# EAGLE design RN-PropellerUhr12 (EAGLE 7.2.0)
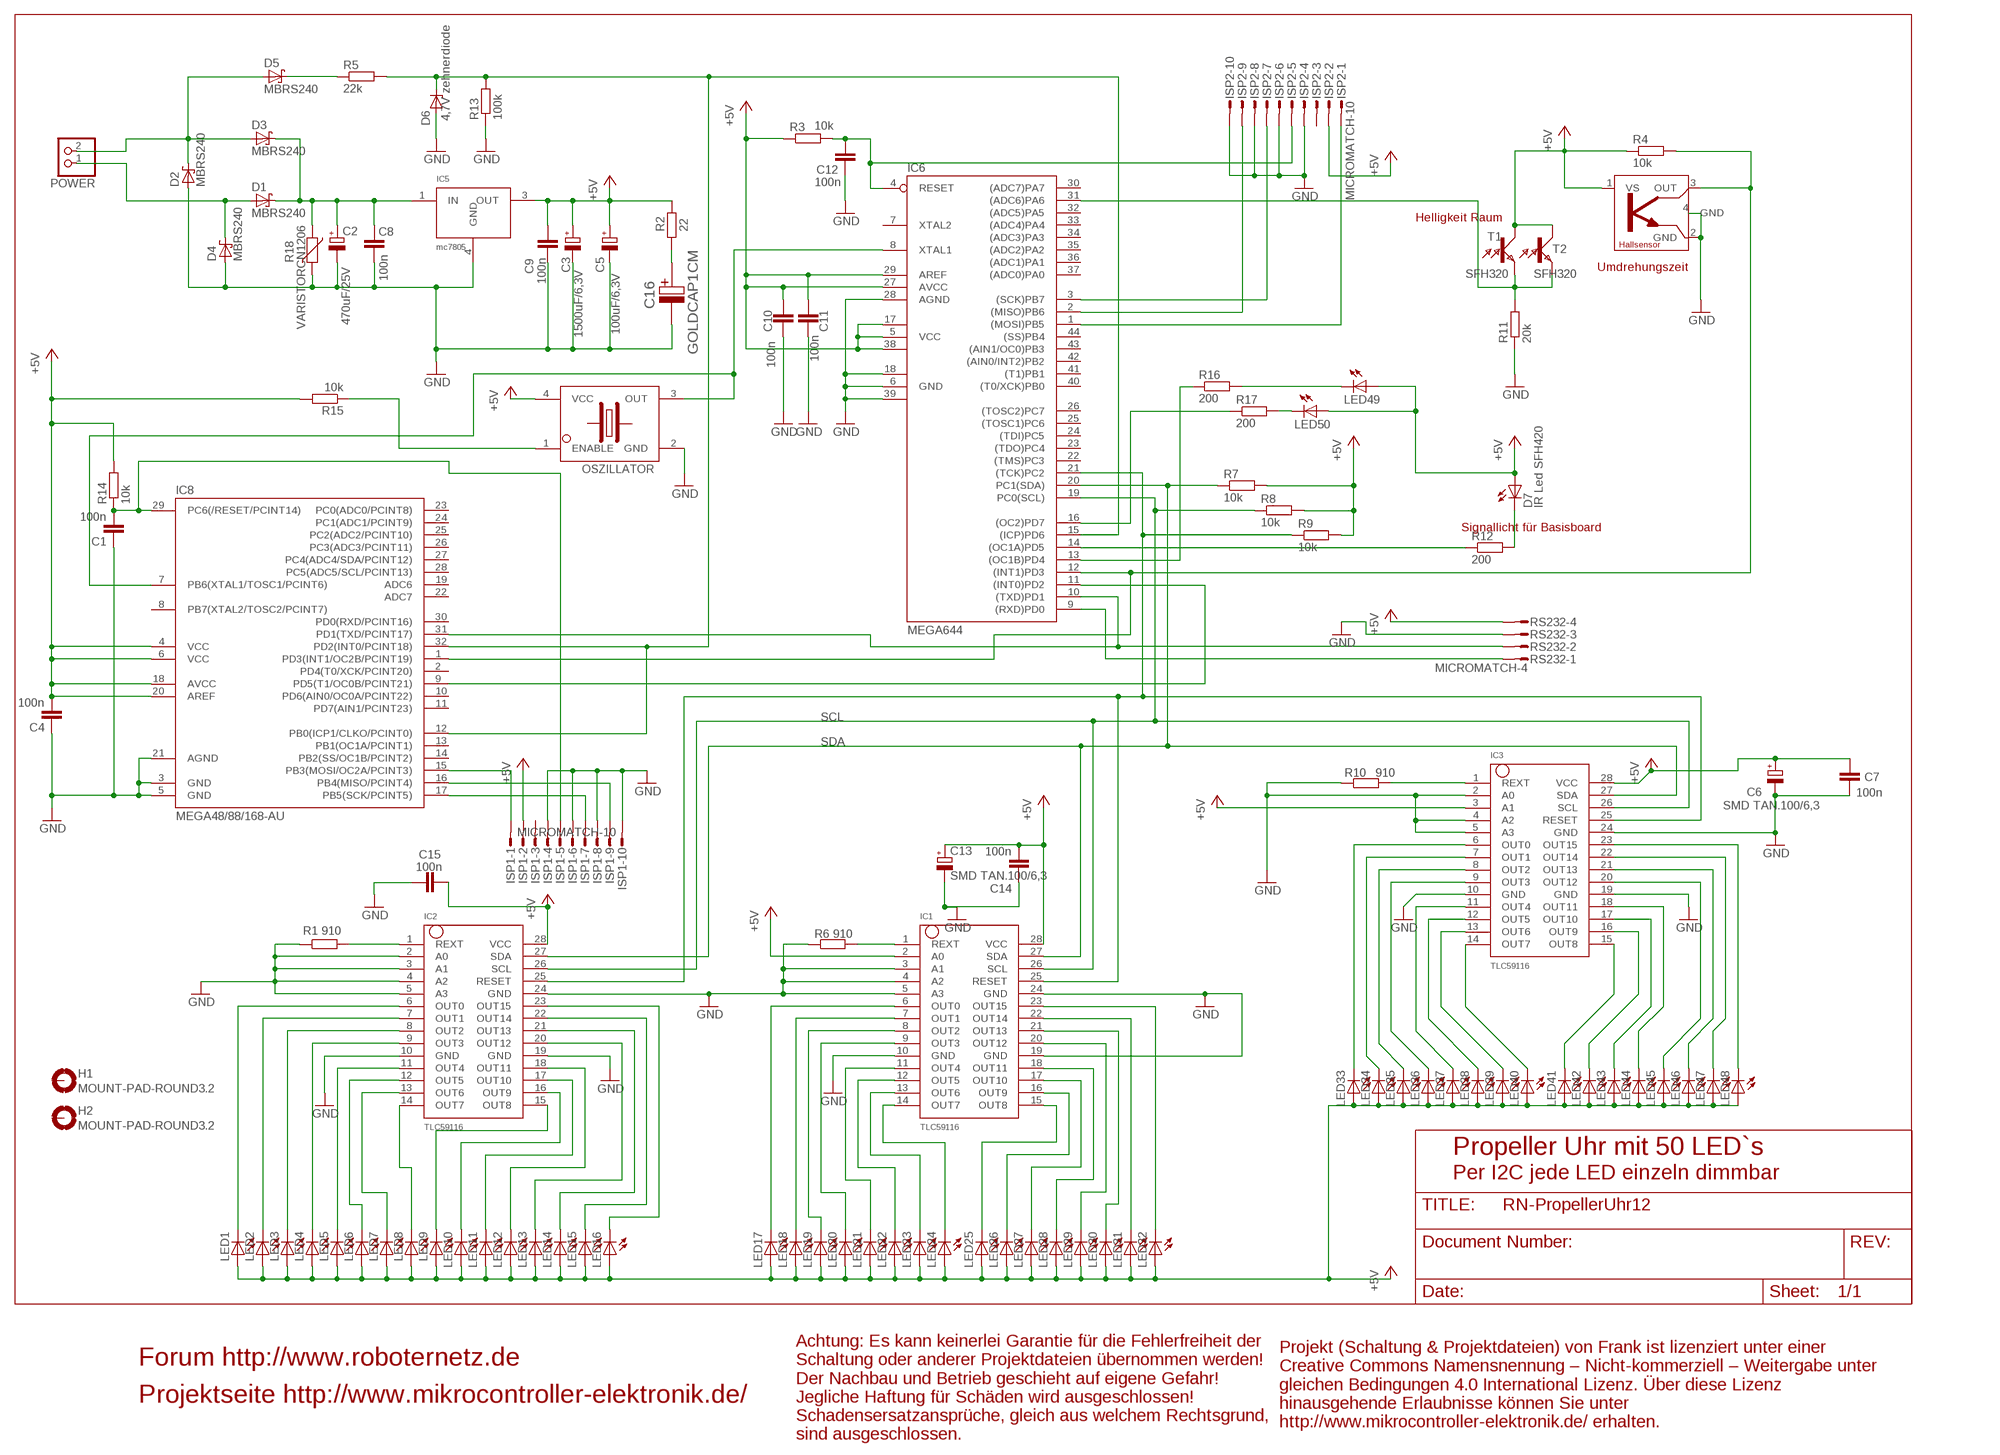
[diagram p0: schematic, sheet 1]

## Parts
C1  100n  C-EUC1206  [C1206]
C2  470uF/25V  CPOL-EU153CLV-1014  [153CLV-1014]
C3  1500uF/6,3V  CPOL-EU153CLV-1014  [153CLV-1014]
C4  100n  C-EUC1206  [C1206]
C5  100uF/6,3V  CPOL-EU153CLV-0605  [153CLV-0605]
C6  SMD TAN.100/6,3  CPOL-EUSMCD  [SMC_D]
C7  100n  C-EUC1206  [C1206]
C8  100n  C-EUC1206  [C1206]
C9  100n  C-EUC1206  [C1206]
C10  100n  C-EUC1206  [C1206]
C11  100n  C-EUC1206  [C1206]
C12  100n  C-EUC1206  [C1206]
C13  SMD TAN.100/6,3  CPOL-EUSMCD  [SMC_D]
C14  100n  C-EUC1206  [C1206]
C15  100n  C-EUC1206  [C1206]
C16  GOLDCAP1CM  [GOLDCAP10MM]
D1  MBRS240  [SMB]
D2  MBRS240  [SMB]
D3  MBRS240  [SMB]
D4  MBRS240  [SMB]
D5  MBRS240  [SMB]
D6  4,7V zehnerdiode  ZENER-DIODESOT23  [SOT23]
D7  IR Led SFH420  SFH420_IRLED  [OSRAM_SFH320]
H1  MOUNT-PAD-ROUND3.2  [3,2-PAD]
H2  MOUNT-PAD-ROUND3.2  [3,2-PAD]
IC1  TLC59116  [PW_R-PDSO-G28]
IC2  TLC59116  [PW_R-PDSO-G28]
IC3  TLC59116  [PW_R-PDSO-G28]
IC5  mc7805  MC7805  [DPAK]
IC6  MEGA644  MEGA32-A  [TQFP44]
IC7  TLE4905  TLE4905SOT89  [SOT89]
IC8  MEGA48/88/168-AU  [TQFP32-08]
ISP1  MICROMATCH-10  [MICROMATCH-10]
ISP2  MICROMATCH-10  [MICROMATCH-10]
LED1  LEDSMT1206  [1206]
LED2  LEDSMT1206  [1206]
LED3  LEDSMT1206  [1206]
LED4  LEDSMT1206  [1206]
LED5  LEDSMT1206  [1206]
LED6  LEDSMT1206  [1206]
LED7  LEDSMT1206  [1206]
LED8  LEDSMT1206  [1206]
LED9  LEDSMT1206  [1206]
LED10  LEDSMT1206  [1206]
LED11  LEDSMT1206  [1206]
LED12  LEDSMT1206  [1206]
LED13  LEDSMT1206  [1206]
LED14  LEDSMT1206  [1206]
LED15  LEDSMT1206  [1206]
LED16  LEDSMT1206  [1206]
LED17  LEDSMT1206  [1206]
LED18  LEDSMT1206  [1206]
LED19  LEDSMT1206  [1206]
LED20  LEDSMT1206  [1206]
LED21  LEDSMT1206  [1206]
LED22  LEDSMT1206  [1206]
LED23  LEDSMT1206  [1206]
LED24  LEDSMT1206  [1206]
LED25  LEDSMT1206  [1206]
LED26  LEDSMT1206  [1206]
LED27  LEDSMT1206  [1206]
LED28  LEDSMT1206  [1206]
LED29  LEDSMT1206  [1206]
LED30  LEDSMT1206  [1206]
LED31  LEDSMT1206  [1206]
LED32  LEDSMT1206  [1206]
LED33  LEDSMT1206  [1206]
LED34  LEDSMT1206  [1206]
LED35  LEDSMT1206  [1206]
LED36  LEDSMT1206  [1206]
LED37  LEDSMT1206  [1206]
LED38  LEDSMT1206  [1206]
LED39  LEDSMT1206  [1206]
LED40  LEDSMT1206  [1206]
LED41  LEDSMT1206  [1206]
LED42  LEDSMT1206  [1206]
LED43  LEDSMT1206  [1206]
LED44  LEDSMT1206  [1206]
LED45  LEDSMT1206  [1206]
LED46  LEDSMT1206  [1206]
LED47  LEDSMT1206  [1206]
LED48  LEDSMT1206  [1206]
LED49  LEDSMT1206  [1206]
LED50  LEDSMT1206  [1206]
OSZILLATOR  OSZILLATOR_AQO7050  [QUARZOSZILLATOR_AQO7050]
POWER  PINHD-1X2  [1X02]
R1  910  R-EU_M1206  [M1206]
R2  22  R-EU_M1206  [M1206]
R3  10k  R-EU_M1206  [M1206]
R4  10k  R-EU_M1206  [M1206]
R5  22k  R-EU_M1206  [M1206]
R6  910  R-EU_M1206  [M1206]
R7  10k  R-EU_M1206  [M1206]
R8  10k  R-EU_M1206  [M1206]
R9  10k  R-EU_M1206  [M1206]
R10  910  R-EU_M1206  [M1206]
R11  20k  R-EU_M1206  [M1206]
R12  200  R-EU_M1206  [M1206]
R13  100k  R-EU_M1206  [M1206]
R14  10k  R-EU_M1206  [M1206]
R15  10k  R-EU_M1206  [M1206]
R16  200  R-EU_M1206  [M1206]
R17  200  R-EU_M1206  [M1206]
R18  VARISTORCN1206  [CT/CN1206]
RS232  MICROMATCH-4  [MICROMATCH-4]
T1  SFH320  [OSRAM_SFH320]
T2  SFH320  [OSRAM_SFH320]

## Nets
+5V [Power]: C3.+ C4.2 C5.+ C6.+ C7.2 C9.2 C10.2 C11.2 C13.+ C14.2 C15.1 D7.E(A) IC1.2(A0) IC1.28(VCC) IC2.28(VCC) IC3.3(A1) IC3.28(VCC) IC5.3(OUT) IC6.5(VCC) IC6.17(VCC1) IC6.27(AVCC) IC6.29(AREF) IC6.38(VCC2) IC7.1(VS) IC8.4(VCC) IC8.6(VCC) IC8.18(AVCC) IC8.20(AREF) ISP1.2 ISP2.2 LED1.A LED2.A LED3.A LED4.A LED5.A LED6.A LED7.A LED8.A LED9.A LED10.A LED11.A LED12.A LED13.A LED14.A LED15.A LED16.A LED17.A LED18.A LED19.A LED20.A LED21.A LED22.A LED23.A LED24.A LED25.A LED26.A LED27.A LED28.A LED29.A LED30.A LED31.A LED32.A LED33.A LED34.A LED35.A LED36.A LED37.A LED38.A LED39.A LED40.A LED41.A LED42.A LED43.A LED44.A LED45.A LED46.A LED47.A LED48.A LED49.A LED50.A OSZILLATOR.4(VCC) R2.2 R3.1 R4.1 R7.2 R8.2 R9.2 R14.2 R15.2 RS232.4 T1.C T2.C
GND [Power]: C1.1 C2.- C3.- C4.1 C5.- C6.- C7.1 C8.1 C9.1 C10.1 C11.1 C12.1 C13.- C14.1 C15.2 C16.M D2.A D4.A D6.1(A) IC1.3(A1) IC1.4(A2) IC1.5(A3) IC1.10(GND) IC1.19(GND) IC1.24(GND) IC2.2(A0) IC2.3(A1) IC2.4(A2) IC2.5(A3) IC2.10(GND) IC2.19(GND) IC2.24(GND) IC3.2(A0) IC3.4(A2) IC3.5(A3) IC3.10(GND) IC3.19(GND) IC3.24(GND) IC5.4(GND) IC6.6(GND) IC6.18(GND1) IC6.28(AGND) IC6.39(GND2) IC7.2(GND) IC7.4(GND) IC8.3(GND) IC8.5(GND) IC8.21(AGND) ISP1.4 ISP1.6 ISP1.8 ISP1.10 ISP2.4 ISP2.6 ISP2.8 ISP2.10 OSZILLATOR.2(GND) R1.1 R6.1 R10.1 R11.1 R13.1 R18.2 RS232.3
N$1 [Power]: D1.A D4.C POWER.1
N$2 [Power]: D2.C D3.A D5.A POWER.2
N$3 [Power]: C2.+ C8.2 D1.C D3.C IC5.1(IN) R18.1
N$5: IC6.8(XTAL1) IC8.7(PB6(XTAL1/TOSC1/PCINT6)) OSZILLATOR.3(OUT)
N$6: IC1.25(RESET) IC2.25(RESET) IC3.25(RESET) IC6.21((TCK)PC2) R9.1
N$7: IC1.14(OUT7) LED24.C
N$8: IC2.1(REXT) R1.2
N$9: C16.P R2.1
N$10: IC1.6(OUT0) LED17.C
N$11: IC6.2((MISO)PB6) ISP2.9
N$12: IC6.3((SCK)PB7) ISP2.7
N$13: IC6.1((MOSI)PB5) ISP2.1
N$14: IC6.12((INT1)PD3) IC7.3(OUT) IC8.1(PD3(INT1/OC2B/PCINT19)) R4.2
N$15: IC1.7(OUT1) LED18.C
N$16: IC1.8(OUT2) LED19.C
N$17: IC1.9(OUT3) LED20.C
N$18: IC1.15(OUT8) LED25.C
N$19: IC1.11(OUT4) LED21.C
N$20: IC1.12(OUT5) LED22.C
N$21: IC1.13(OUT6) LED23.C
N$22: IC1.16(OUT9) LED26.C
N$23: IC1.17(OUT10) LED27.C
N$24: IC1.18(OUT11) LED28.C
N$25: IC1.20(OUT12) LED29.C
N$26: IC1.21(OUT13) LED30.C
N$27: IC1.22(OUT14) LED31.C
N$28: IC1.23(OUT15) LED32.C
N$29: IC1.1(REXT) R6.2
N$30: D6.3(C) IC6.15((ICP)PD6) IC8.12(PB0(ICP1/CLKO/PCINT0)) IC8.32(PD2(INT0/PCINT18)) R5.2 R13.2
N$31: D5.C R5.1
N$33: C1.2 IC8.29(PC6(/RESET/PCINT14)) ISP1.5 R14.1
N$34: IC3.6(OUT0) LED33.C
N$35: IC3.7(OUT1) LED34.C
N$36: IC3.8(OUT2) LED35.C
N$37: IC3.9(OUT3) LED36.C
N$38: IC3.11(OUT4) LED37.C
N$39: IC3.12(OUT5) LED38.C
N$40: IC3.13(OUT6) LED39.C
N$41: IC2.6(OUT0) LED1.C
N$42: IC2.7(OUT1) LED2.C
N$43: IC2.8(OUT2) LED3.C
N$44: IC2.9(OUT3) LED4.C
N$45: IC2.11(OUT4) LED5.C
N$46: IC2.12(OUT5) LED6.C
N$47: IC2.13(OUT6) LED7.C
N$48: IC2.14(OUT7) LED8.C
N$49: IC2.15(OUT8) LED9.C
N$50: IC2.16(OUT9) LED10.C
N$51: IC2.17(OUT10) LED11.C
N$52: IC2.18(OUT11) LED12.C
N$53: IC2.20(OUT12) LED13.C
N$54: IC2.21(OUT13) LED14.C
N$55: IC2.22(OUT14) LED15.C
N$56: IC2.23(OUT15) LED16.C
N$57: C12.2 IC6.4(RESET) ISP2.5 R3.2
N$58: IC3.14(OUT7) LED40.C
N$59: IC3.15(OUT8) LED41.C
N$60: IC3.16(OUT9) LED42.C
N$61: IC3.17(OUT10) LED43.C
N$62: IC3.18(OUT11) LED44.C
N$63: IC3.20(OUT12) LED45.C
N$64: IC3.21(OUT13) LED46.C
N$65: IC3.22(OUT14) LED47.C
N$66: IC3.23(OUT15) LED48.C
N$67: IC3.1(REXT) R10.2
N$68: IC6.31((ADC6)PA6) R11.2 T1.E T2.E
N$69: D7.C R12.2
N$70: IC6.14((OC1A)PD5) R12.1
N$71: IC8.15(PB3(MOSI/OC2A/PCINT3)) ISP1.1
N$72: OSZILLATOR.1(ENABLE) R15.1
N$73: IC8.17(PB5(SCK/PCINT5)) ISP1.7
N$74: IC8.16(PB4(MISO/PCINT4)) ISP1.9
N$75: LED50.C R17.2
N$76: LED49.C R16.2
N$77: IC6.16((OC2)PD7) R17.1
N$78: IC6.13((OC1B)PD4) R16.1
N$79: IC6.11((INT0)PD2) IC8.9(PD5(T1/OC0B/PCINT21))
RXD: IC6.9((RXD)PD0) RS232.1
SCL: IC1.26(SCL) IC2.26(SCL) IC3.26(SCL) IC6.19(PC0(SCL)) R8.1
SDA: IC1.27(SDA) IC2.27(SDA) IC3.27(SDA) IC6.20(PC1(SDA)) R7.1
TXD: IC6.10((TXD)PD1) IC8.31(PD1(TXD/PCINT17)) RS232.2
Unconnected: H1.B3,2(MOUNT) H2.B3,2(MOUNT) IC6.7(XTAL2) IC6.22((TMS)PC3) IC6.23((TDO)PC4) IC6.24((TDI)PC5) IC6.25((TOSC1)PC6) IC6.26((TOSC2)PC7) IC6.30((ADC7)PA7) IC6.32((ADC5)PA5) IC6.33((ADC4)PA4) IC6.34((ADC3)PA3) IC6.35((ADC2)PA2) IC6.36((ADC1)PA1) IC6.37((ADC0)PA0) IC6.40((T0/XCK)PB0) IC6.41((T1)PB1) IC6.42((AIN0/INT2)PB2) IC6.43((AIN1/OC0)PB3) IC6.44((SS)PB4) IC8.2(PD4(T0/XCK/PCINT20)) IC8.8(PB7(XTAL2/TOSC2/PCINT7)) IC8.10(PD6(AIN0/OC0A/PCINT22)) IC8.11(PD7(AIN1/PCINT23)) IC8.13(PB1(OC1A/PCINT1)) IC8.14(PB2(SS/OC1B/PCINT2)) IC8.19(ADC6) IC8.22(ADC7) IC8.23(PC0(ADC0/PCINT8)) IC8.24(PC1(ADC1/PCINT9)) IC8.25(PC2(ADC2/PCINT10)) IC8.26(PC3(ADC3/PCINT11)) IC8.27(PC4(ADC4/SDA/PCINT12)) IC8.28(PC5(ADC5/SCL/PCINT13)) IC8.30(PD0(RXD/PCINT16)) ISP1.3 ISP2.3

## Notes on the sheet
- Helligkeit Raum
- Umdrehungszeit
- Signallicht für Basisboard
- Propeller Uhr mit 50 LED`s
- Per I2C jede LED einzeln dimmbar
- Forum http://www.roboternetz.de
- Projektseite http://www.mikrocontroller-elektronik.de/
- Projekt (Schaltung & Projektdateien) von Frank ist lizenziert unter einer
  Creative Commons Namensnennung – Nicht-kommerziell – Weitergabe unter
  gleichen Bedingungen 4.0 International Lizenz. Über diese Lizenz
  hinausgehende Erlaubnisse können Sie unter
  http://www.mikrocontroller-elektronik.de/ erhalten.
- Achtung: Es kann keinerlei Garantie für die Fehlerfreiheit der
  Schaltung oder anderer Projektdateien übernommen werden!
  Der Nachbau und Betrieb geschieht auf eigene Gefahr! 
  Jegliche Haftung für Schäden wird ausgeschlossen!
  Schadensersatzansprüche, gleich aus welchem Rechtsgrund,
  sind ausgeschlossen.

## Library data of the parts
C1 C4 C7-C12 C14 C15 = rcl:C-EU: CAPACITOR, European symbol
C2 C3 = resistor:CPOL-EU: POLARIZED CAPACITOR, European symbol
C5 C6 C13 = rcl:CPOL-EU: POLARIZED CAPACITOR, European symbol
C16 = RoboterNetzNeu:GOLDCAP1CM: Goldcap (z.B. 100000uF 10V)
D1-D5 = RoboterNetzNeu:MBRS240: Schottky Power Rectifier
D6 = diode:ZENER-DIODE: Z-Diode
D7 = RoboterNetzNeu:SFH420_IRLED: Infrarot Diode SFH420
H1 H2 = holes:MOUNT-PAD-ROUND: MOUNTING PAD, round
IC1-IC3 = RoboterNetzNeu:TLC59116: I2C LED Treiber 16 fach (mit Helligkeitsregelung) Bezug Robotikhardware.de
IC5 = RoboterNetzNeu:MC7805: 1 A Spannungsregler im DPAK2 Gehäuse
IC6 = atmel:MEGA32: MICROCONTROLLER 32 Kbytes FLASH 2 Kbytes SRAM 1 Kbytes EEPROM USART 8-channel 10 bit ADC Source: www.atmel.com .. doc2503.pdf
IC7 = RoboterNetzNeu:TLE4905: Hallsensor / Bezug Robotikhardware.de
IC8 = avr-4:MEGA48/88/168
ISP1 ISP2 = con-amp-micromatch:MICROMATCH-10: MicroMaTch 10 8-215464-0 / 1-215464-0 Drawing Number C-215464 DDEController.pdf
LED1-LED50 = led:LED: LED
OSZILLATOR = RoboterNetzNeu:OSZILLATOR_AQO7050: Quarzoszillator AQO7050 5V http://www.buerklin.com/
POWER = pinhead:PINHD-1X2: PIN HEADER
R1-R17 = rcl:R-EU_: RESISTOR, European symbol
R18 = varistor:VARISTOR: VARISTOR
RS232 = con-amp-micromatch:MICROMATCH-4: MicroMaTch 4 7-215464-4 / 0-215464-4 Drawing Number C-215464 DDEController.pdf
T1 T2 = RoboterNetzNeu:SFH320: Fototransistor

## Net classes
0 default: width 0.406 mm
1 Power: width 0.406 mm

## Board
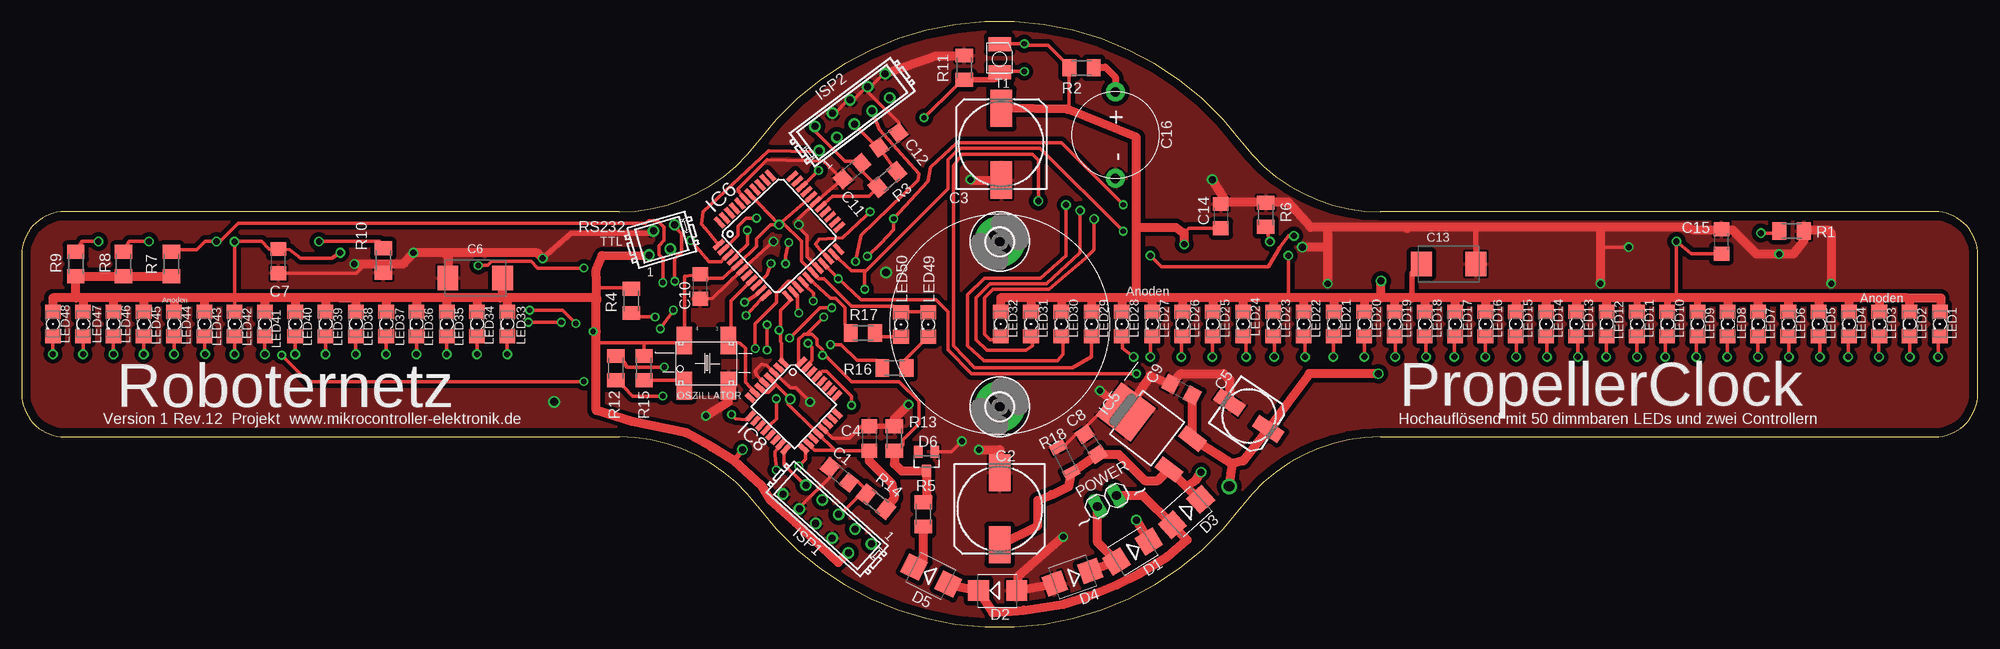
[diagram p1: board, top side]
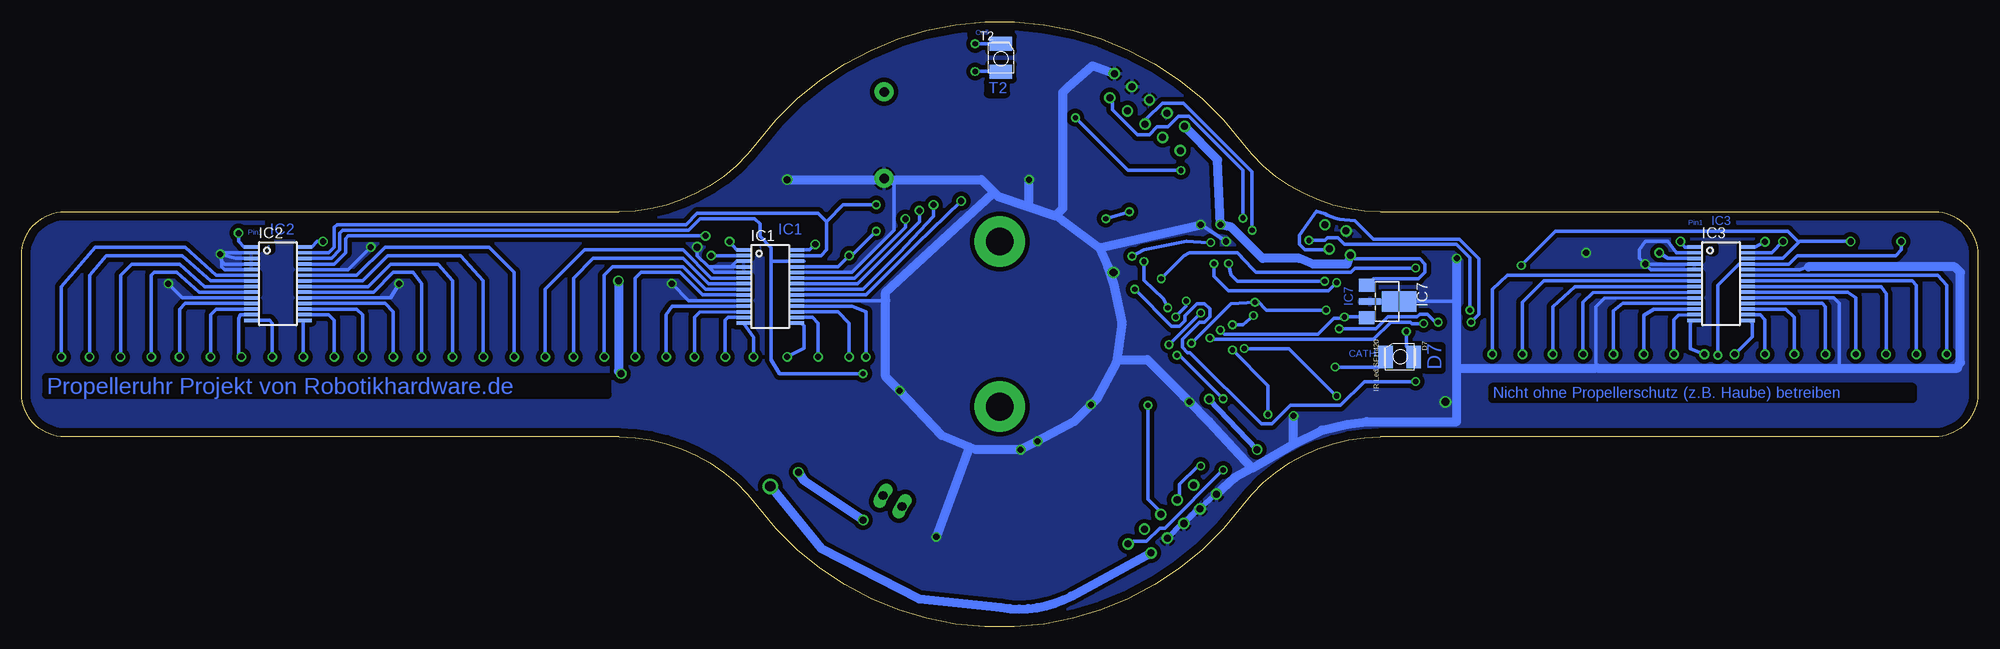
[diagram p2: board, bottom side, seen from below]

Size 226 x 69.92 mm. Coordinates in mm from the lower left corner, seen from the top.
Outline: 141,55.96 arc106 85,55.96
Outline: 141,13.96 arc-106 85,13.96 arc53 69,21.96 5,21.96 arc-90 0,26.96 0,42.96 arc-90 5,47.96 69,47.96 arc53 85,55.96
Outline: 141,13.96 arc-53 157,21.96 221,21.96 arc90 226,26.96 226,42.96 arc90 221,47.96 157,47.96 arc-53 141,55.96
Copper layers (1*16): Top 0.035mm / dielectric 1.5mm / Bottom 0.035mm
Design rules "default *": minimum track width 12mil, minimum drill 24mil, track to track 8mil, track to pad 8mil, pad to pad 8mil, via to via 14mil, smd to smd 9mil, copper to edge 40mil, drill to drill 8mil, minimum pad ring 10mil, minimum via ring 8mil, stop-mask expansion 4mil, vias tented up to drill 0mil, thermal gap 10mil
tRestrict: area 77.8,27.3 to 80.4,34.1

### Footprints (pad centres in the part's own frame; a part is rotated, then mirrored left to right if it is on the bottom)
C1206 = smd 1.6 x 1.8: 1 -1.4,0; 2 1.4,0
153CLV-1014 = smd 4.3 x 2.5: + 4.15,0; - -4.15,0
153CLV-0605 = smd 3.5 x 1.6: + 2.7,0; - -2.7,0
SMC_D = smd 2.4 x 2.8: + -3.15,0; - 3.15,0
GOLDCAP10MM = drill 1.1 pad 2.184: M 5,0; P -5,0
SMB = smd 2.4 x 2.4: A 2.2,0; C -2.2,0
SOT23 = smd 1 x 1.4: 1 -0.95,-1.1; 2 0.95,-1.1; 3 0,1.1
OSRAM_SFH320 = smd 2.6 x 1.65: C 0,-1.62; E 0,1.62
3,2-PAD = drill 3.2 pad 5.842: B3,2 0,0
PW_R-PDSO-G28 = smd 0.4 x 1.6: 1 -4.225,-3.1; 2 -3.575,-3.1; 3 -2.925,-3.1; 4 -2.275,-3.1; 5 -1.625,-3.1; 6 -0.975,-3.1; 7 -0.325,-3.1; 8 0.325,-3.1; 9 0.975,-3.1; 10 1.625,-3.1; 11 2.275,-3.1; 12 2.925,-3.1; 13 3.575,-3.1; 14 4.225,-3.1; 15 4.225,3.1; 16 3.575,3.1; 17 2.925,3.1; 18 2.275,3.1; 19 1.625,3.1; 20 0.975,3.1; 21 0.325,3.1; 22 -0.325,3.1; 23 -0.975,3.1; 24 -1.625,3.1; 25 -2.275,3.1; 26 -2.925,3.1; 27 -3.575,3.1; 28 -4.225,3.1
DPAK = smd 1.6 x 2.997: 1 -2.261,-4.928; 3 2.21,-4.928 | smd 4.826 x 5: 4 0,3.053
TQFP44 = smd 1.5 x 0.5: 1 -5.8,4; 2 -5.8,3.2; 3 -5.8,2.4; 4 -5.8,1.6; 5 -5.8,0.8; 6 -5.8,0; 7 -5.8,-0.8; 8 -5.8,-1.6; 9 -5.8,-2.4; 10 -5.8,-3.2; 11 -5.8,-4; 23 5.8,-4; 24 5.8,-3.2; 25 5.8,-2.4; 26 5.8,-1.6; 27 5.8,-0.8; 28 5.8,0; 29 5.8,0.8; 30 5.8,1.6; 31 5.8,2.4; 32 5.8,3.2; 33 5.8,4 | smd 0.5 x 1.5: 12 -4,-5.8; 13 -3.2,-5.8; 14 -2.4,-5.8; 15 -1.6,-5.8; 16 -0.8,-5.8; 17 0,-5.8; 18 0.8,-5.8; 19 1.6,-5.8; 20 2.4,-5.8; 21 3.2,-5.8; 22 4,-5.8; 34 4,5.8; 35 3.2,5.8; 36 2.4,5.8; 37 1.6,5.8; 38 0.8,5.8; 39 0,5.8; 40 -0.8,5.8; 41 -1.6,5.8; 42 -2.4,5.8; 43 -3.2,5.8; 44 -4,5.8
SOT89 = smd 1.5 x 1.8: 1 -1.9,-2.1; 3 1.9,-2.1 | smd 0.7 x 2.55: 2 0,-1.73 | smd 2.4 x 4: 4 0,1.652
TQFP32-08 = smd 1.27 x 0.559: 1 -4.293,2.8; 2 -4.293,2; 3 -4.293,1.2; 4 -4.293,0.4; 5 -4.293,-0.4; 6 -4.293,-1.2; 7 -4.293,-2; 8 -4.293,-2.8; 17 4.293,-2.8; 18 4.293,-2; 19 4.293,-1.2; 20 4.293,-0.4; 21 4.293,0.4; 22 4.293,1.2; 23 4.293,2; 24 4.293,2.8 | smd 0.559 x 1.27: 9 -2.8,-4.293; 10 -2,-4.293; 11 -1.2,-4.293; 12 -0.4,-4.293; 13 0.4,-4.293; 14 1.2,-4.293; 15 2,-4.293; 16 2.8,-4.293; 25 2.8,4.293; 26 2,4.293; 27 1.2,4.293; 28 0.4,4.293; 29 -0.4,4.293; 30 -1.2,4.293; 31 -2,4.293; 32 -2.8,4.293
MICROMATCH-10 = drill 0.813: 1 5.715,1.27; 2 4.445,-1.27; 3 3.175,1.27; 4 1.905,-1.27; 5 0.635,1.27; 6 -0.635,-1.27; 7 -1.905,1.27; 8 -3.175,-1.27; 9 -4.445,1.27; 10 -5.715,-1.27
1206 = smd 1.6 x 1.803: A -1.422,0; C 1.422,0
QUARZOSZILLATOR_AQO7050 = smd 1.8 x 3.2: 1 -2.857,-2.723; 2 2.223,-2.723; 3 2.223,2.505; 4 -2.857,2.505
1X02 = drill 1.016 long: 1 -1.27,0; 2 1.27,0
M1206 = smd 1.6 x 2: 1 -1.4,0; 2 1.4,0
CT/CN1206 = smd 1.2 x 1.8: 1 -1.65,0; 2 1.65,0
MICROMATCH-4 = drill 0.813: 1 1.905,1.27; 2 0.635,-1.27; 3 -0.635,1.27; 4 -1.905,-1.27

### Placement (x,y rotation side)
C1  94.49,17.57 321.3 top
C2  112.99,13.65 270 top
C3  113.19,55.77 90 top
C4  97.91,21.77 270 top
C5  141.78,24.39 325.8 top
C6  52.41,40.3 180 top
C7  29.66,42.25 90 top
C8  123.57,21.11 303.1 top
C9  134,27.4 332.3 top
C10  78.41,39.32 90 top
C11  95.96,52.65 40.3 top
C12  100.18,56.22 217 top
C13  164.86,41.92 0 top
C14  138.53,47.45 270 top
C15  196.38,44.52 90 top
C16  126.36,56.81 270 top
D1  128.36,8.72 211.6 top
D2  112.75,4.21 0 top
D3  134.58,13.27 222 top
D4  121.41,5.75 199.7 top
D5  105.07,5.94 333.4 top
D6  104.54,19.12 180 top
D7  66.81,31.19 270 bottom
H1  113,25.44 0 top
H2  113,44.51 0 top
IC1  139.51,39.32 270 bottom
IC2  196.38,39.65 270 bottom
IC3  29.66,39.65 270 bottom
IC5  130.02,22.98 52.7 top
IC6  87.51,45.17 42.8 top
IC7  68.5,37.59 270 bottom
IC8  89.2,25.55 316.4 top
ISP1  93.07,12.47 318.1 top
ISP2  95.96,59.47 216.9 top
LED1  221.61,35 270 top
LED2  218.11,35 270 top
LED3  214.61,35 270 top
LED4  211.11,35 270 top
LED5  207.61,35 270 top
LED6  204.11,35 270 top
LED7  200.61,35 270 top
LED8  197.11,35 270 top
LED9  193.61,35 270 top
LED10  190.11,35 270 top
LED11  186.61,35 270 top
LED12  183.11,35 270 top
LED13  179.61,35 270 top
LED14  176.11,35 270 top
LED15  172.61,35 270 top
LED16  169.11,35 270 top
LED17  165.61,35 270 top
LED18  162.11,35 270 top
LED19  158.61,35 270 top
LED20  155.11,35 270 top
LED21  151.61,35 270 top
LED22  148.11,35 270 top
LED23  144.61,35 270 top
LED24  141.11,35 270 top
LED25  137.61,35 270 top
LED26  134.11,35 270 top
LED27  130.61,35 270 top
LED28  127.11,35 270 top
LED29  123.61,35 270 top
LED30  120.11,35 270 top
LED31  116.61,35 270 top
LED32  113.11,35 270 top
LED33  56.11,35 270 top
LED34  52.61,35 270 top
LED35  49.11,35 270 top
LED36  45.61,35 270 top
LED37  42.11,35 270 top
LED38  38.61,35 270 top
LED39  35.11,35 270 top
LED40  31.61,35 270 top
LED41  28.11,35 270 top
LED42  24.61,35 270 top
LED43  21.11,35 270 top
LED44  17.61,35 270 top
LED45  14.11,35 270 top
LED46  10.61,35 270 top
LED47  7.11,35 270 top
LED48  3.61,35 270 top
LED49  104.73,34.94 270 top
LED50  101.6,34.94 270 top
OSZILLATOR  79.42,30.59 0 top
POWER  125.4,14.55 29.7 top
R1  204.48,45.73 180 top
R2  122.45,64.58 180 top
R3  100.02,51.68 39.9 top
R4  70.42,37.67 270 top
R5  104.17,13.01 90 top
R6  143.73,47.61 270 top
R7  17.31,41.92 270 top
R8  11.78,41.92 270 top
R9  6.26,41.92 270 top
R10  41.78,42.33 90 top
R11  108.9,64.6 270 top
R12  68.66,29.9 90 top
R13  100.83,21.77 270 top
R14  98.71,14.47 322 top
R15  71.91,29.9 90 top
R16  100.83,29.9 0 top
R17  97.19,33.96 0 top
R18  120.5,19.29 117.6 top
RS232  73.96,44.71 16.2 top
T1  112.99,65.69 180 top
T2  112.88,65.74 180 bottom

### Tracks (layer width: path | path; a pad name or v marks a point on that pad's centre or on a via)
+5V  (via drill 0.61, 0.7, 0.8, 1.2)
  Top 0.406: 191.18,38.02 v191.18,44.52 192.91,43.12 C15.1 | 146.33,38.02 v146.33,42.9 | 24.61,38.4 LED42.A | 24.61,38.4 v24.61,44.5 24.63,44.52 27.71,44.52 28.58,43.65 C7.2 30.96,43.55 32.26,42.57 35.83,42.57 v36.81,43.22 | LED42.A | C14.2 134.86,46.05 134.31,45.5 | 93.83,20.51 93.96,20.37 C4.2 | 93.83,20.51 IC8.20 91.61,22.71 88.56,25.75 v88.81,26.32 87.16,28 | 71.91,32.82 R15.2 | C10.2 76.56,40.51 OSZILLATOR.4 arc90 76.5,32.82 71.91,32.82 | 66.38,32.82 71.91,32.82 | 86.53,28.6 IC8.4 87.16,28 | v87.51,46.47 IC6.38 | v87.51,46.47 87.88,46.8 | 87.88,46.8 IC6.29 | IC6.27 93.68,49.72 97.88,49.72 R3.1 97.02,52.7 C11.2 96.03,53.8 95.12,53.8 91.77,57.15 ISP2.2 | RS232.4 70.42,43.11 | 82.79,41.89 81.01,40.3 78.08,40.3 | T1.C 114.17,67.36 v115.84,67.36 116.3,67.21 118.59,67.21 120.26,65.53 R2.2 121.03,63.7 121.03,60.2 120.85,59.77 | LED49.A 103.96,36.42 102.43,36.42 LED50.A 100.76,37.03 95.88,37.03 92.68,40.23 92.07,40.23 91.92,40.38 IC6.17 90.11,42.26 90.11,44.52 87.88,46.75 87.88,46.8 | IC8.18 91.31,20.72 91.61,20.42 93.75,20.42 93.83,20.51 | IC8.6 85.67,27.28 85.82,27.13 86.28,27.13 87.04,27.89 87.16,28 | IC6.5 82.77,41.91 82.79,41.89 | R4.1 69.52,39.17 66.41,39.17 | 66.38,34.14 v66.01,34.14 | 24.61,38.4 24.56,38.4 24.56,38 | 82.79,41.89 84.91,44 84.91,44.85 86.53,46.47 v87.51,46.47
  Top 0.61: 160.63,38.02 160.63,40.85 C13.+ | 82.31,19.17 v83.28,20.47
  Top 0.813: 169.08,38.02 169.11,38 | 221.73,36.55 LED1.A | 172.66,38.02 172.61,37.97 | 176.23,38.02 176.11,37.9 | 179.81,38.02 179.61,37.82 | 183.06,38.02 183.11,37.97 | LED11.A 186.61,38 186.63,38.02 | LED10.A 190.11,37.92 191.18,38.02 | LED9.A 193.61,37.87 193.46,38.02 | 197.03,38.02 197.11,37.95 | 207.76,38.02 207.61,37.87 | 211.33,38.02 211.11,37.8 | 214.26,38.02 214.61,37.67 | LED2.A 218.13,36.42 218.16,36.4 | 218.16,37.7 217.83,38.02 | 116.76,38.02 116.61,38.02 | 120.01,38.02 120.11,38.02 | 123.58,38.02 123.61,38.02 | 126.83,38.02 127.11,38.02 | 133.98,38.02 134.11,38.02 | 137.56,38.02 137.61,38.02 | 141.13,38.02 141.11,38.02 | 144.71,38.02 144.61,38.02 | 147.96,38.02 148.11,38.02 | 151.86,38.02 151.61,38.02 | 158.68,38.02 158.61,38.02 | 161.93,38.02 162.11,38.02 | 165.51,38.02 165.61,38.02 | LED35.A 49.53,36.42 49.61,36.5 | LED46.A 11.03,36.42 11.11,36.5 11.11,36 10.61,36.5 | 200.61,38.02 | 155.11,38.02 | 56.11,38 | 52.61,38 | 49.11,38 | 45.61,38 | 42.11,38 | 38.61,38 | 35.11,38 | 31.61,38 | 28.11,38
  Top 1.016: 169.11,38 LED16.A | 204.18,38.02 207.76,38.02 211.33,38.02 214.26,38.02 217.83,38.02 221.73,38.02 221.73,36.55 | 204.18,38.02 200.61,38.02 | 200.61,38.02 197.03,38.02 193.46,38.02 191.18,38.02 186.63,38.02 183.06,38.02 179.81,38.02 177.86,38.02 | 177.86,38.02 176.23,38.02 172.66,38.02 169.08,38.02 165.51,38.02 161.93,38.02 160.63,38.02 158.68,38.02 157.06,38.02 | 172.61,37.97 LED15.A | 176.11,37.9 LED14.A | 179.61,37.82 LED13.A | 183.11,37.97 LED12.A | 197.11,37.95 LED8.A | 200.61,38.02 LED7.A | LED6.A 204.11,37.95 204.18,38.02 | 207.61,37.87 LED5.A | 211.11,37.8 LED4.A | 214.61,37.67 LED3.A | 218.16,36.4 218.16,37.7 | LED32.A 113.11,38.02 116.76,38.02 120.01,38.02 123.58,38.02 126.83,38.02 128.78,38.02 | 157.06,38.02 155.11,38.02 | 155.11,38.02 151.86,38.02 147.96,38.02 146.33,38.02 144.71,38.02 141.13,38.02 137.56,38.02 133.98,38.02 130.08,38.02 | 130.08,38.02 128.78,38.02 | 116.61,38.02 LED31.A | 120.11,38.02 LED30.A | 123.61,38.02 LED29.A | 127.11,38.02 LED28.A | LED27.A 130.61,38.02 130.08,38.02 | 134.11,38.02 LED26.A | 137.61,38.02 LED25.A | 141.11,38.02 LED24.A | 144.61,38.02 LED23.A | 148.11,38.02 LED22.A | 151.61,38.02 LED21.A | 155.11,38.02 LED20.A | 158.61,38.02 LED19.A | 162.11,38.02 LED18.A | 165.61,38.02 LED17.A | v134.31,44.2 134.31,45.5 133.33,46.15 128.78,46.15 | 128.78,38.02 128.78,46.15 | LED48.A 3.61,38 6.26,38 | 7.11,38 6.26,38 | 10.61,38 7.11,38 | 14.11,38 10.61,38 | 17.61,38 14.11,38 | 21.11,38 17.61,38 | 28.11,38 24.56,38 21.11,38 | 31.61,38 28.11,38 | 35.11,38 31.61,38 | 36.81,38 35.11,38 | 36.81,38 38.61,38 LED38.A | 42.11,38 36.81,38 | 45.61,38 42.11,38 | 49.11,38 45.61,38 | 52.61,38 49.11,38 | 55.33,38 52.61,38
  Top 1.016: 56.11,38 55.33,38 | 56.11,38 LED33.A | 52.61,38 LED34.A | 49.11,38 LED35.A | 45.61,38 LED36.A | 42.11,38 LED37.A | 35.11,38 LED39.A | 31.61,38 LED40.A | 28.11,38 LED41.A | 21.11,38 LED43.A | 17.61,38 LED44.A | 14.11,38 LED45.A | 10.61,38 10.61,36.5 | 7.11,38 LED47.A | 177.86,38.02 | C6.+ 55.56,38.22 55.33,38 | 139.81,18.85 IC5.3 135.28,26.75 C9.2 | 139.81,18.85 141.13,19.17 142.39,20.76 C5.+ 148.77,29.25 v156.73,29.25 | 157.06,38.02 v157.06,39.97 | C4.2 97.91,19.17 100.51,16.57 100.83,14.95 R14.2 | 66.41,38 56.11,38 | ISP1.2 94.33,7.47 89.46,12.02 86.53,14.62 85.56,16.25 82.31,19.17 79.71,20.8 76.78,22.42 70.61,23.72 66.38,25.02 66.38,32.82 66.38,34.14 66.38,37.7 arc90 66.41,38 | T1.C 113.04,67.27 | 6.26,38 R9.2 R8.2 R7.2 | 128.78,46.15 128.78,56.55 120.85,59.77 120.79,59.8 C3.+ | 66.41,38 66.41,39.17 66.41,39.67 66.38,41.27 67.03,42.9 RS232.4 | 139.81,18.85 v139.51,16.25
  Bottom 0.406: IC2.28 192.48,43.87 191.83,44.52 v191.18,44.52 | IC1.28 134.96,43.55 v134.31,44.2 | IC3.28 25.76,43.87 v24.61,44.5 | IC3.3 35.83,42.57 v36.81,43.22 | v146.33,42.9 IC1.2 | v115.84,67.36 114.17,67.36 T2.C | IC7.1 69.82,40.23 64.64,40.23 63.88,40.99 63.88,41.91 64.49,42.52 71.95,42.52 RS232.4 | v66.01,34.14 66.01,32.46 D7.E
  Bottom 0.61: v83.28,20.47 v88.81,26.32
  Bottom 1.016: v156.73,29.25 157.06,29.57 v157.06,39.97 | ISP1.2 104.73,3.57 arc39 112.86,2.27 122.28,3.25 133.66,9.1 v139.51,16.25 | ISP2.2 87.83,53.95 v87.51,46.47 86.21,46.15 82.63,42.57 78.41,42.57 76.78,41.92 72.88,41.92 RS232.4
GND  (via drill 0.7, 0.8, 0.9)
  Top 0.406: 182.41,43.87 v185.66,43.87 | 41.79,41.92 R10.1 | C7.1 38.66,40.85 39.73,41.92 | C14.1 138.43,48.85 138.21,49.07 | IC8.21 93.69,21.77 95.63,21.77 96.93,23.07 97.81,23.07 C4.1 | v108.63,21.45 107.41,20.22 D6.1 | C10.1 79.8,37.95 IC6.6 v86.86,44.52 | v91.08,26 90.11,26.97 89.46,27.62 88.81,27.62 IC8.3 86.07,30.24 85.5,30.35 84.73,29.58 84.89,29.1 IC8.5 | ISP2.4 94.2,59.59 95.27,60.65 ISP2.6 96.34,61.11 97.25,62.03 ISP2.8 | C12.1 101.37,58.22 97.86,61.72 ISP2.8 | R18.2 120.57,21.03 121.79,22.25 C8.1 123.16,23.32 124.23,24.38 IC5.4 | IC6.39 82.92,50.17 82.77,50.61 86.12,53.96 92.68,53.8 94.2,52.27 C11.1 IC6.28 89.78,47.12 v89.78,46.47 89.78,46.15 90.76,45.17 90.76,42.74 IC6.18 | C1.1 93.44,17.37 90.24,14.17 ISP1.8 | C15.2 196.46,46.02 196.48,45.82 | ISP2.8 98.32,62.63 99.23,63.55 ISP2.10
  Top 0.61: C13.- 168.01,46.05 168.11,46.15 | R13.1 C4.1 | v60.21,42.57 63.46,45.5 72.74,45.5 arc90 RS232.3
  Top 0.813: 182.73,46.15 182.41,46.15
  Top 1.016: 182.41,46.15 182.41,43.87 v182.41,39.65 | 150.88,46.15 150.88,43.87 | 159.98,46.15 150.88,46.15 | 159.98,46.15 168.11,46.15 182.73,46.15 192.48,46.15 193.13,45.82 196.48,45.82 197.68,45.82 200.44,43.07 v203.04,43.07 204.67,43.07 205.88,44.59 R1.1 205.97,45.82 208.73,45.82 209.06,45.5 v209.06,39.65 | 150.88,43.87 v147.96,43.87 | 150.88,43.87 v150.88,39.65 | 144.06,49.07 139.18,49.07 | 139.18,49.07 138.21,49.07 | 144.06,49.07 146.33,49.07 148.93,46.15 150.88,46.15 | 48.83,43.22 59.56,43.22 v60.21,42.57 | 48.83,43.22 v45.26,43.22 44.07,41.92 42.33,41.92 41.79,41.92 39.73,41.92 v38.43,41.92 | 144.06,49.07 R6.1 | C6.- 49.26,42.8 48.83,43.22 | 159.98,46.15 160.08,46.05 | C3.- 109.66,51.62 v109.61,51.67 | R13.1 100.83,24.05 v102.46,25.67 | v124.56,27.3 126.69,25.67 IC5.4 130.39,29.03 C9.1 133.95,29.25 138.86,29.25 139.55,28.56 C5.- | v110.58,20.47 112.99,20.47 C2.- | D4.A D2.A 115.13,5.85 v120.33,10.4 | v79.06,24.37 81.66,26 OSZILLATOR.2 | R11.1 107.33,65.97 105.71,65.97 ISP2.10 | 139.18,49.07 v137.56,51.67
  Bottom 0.406: IC2.19 183.38,38.02 v182.41,39.65 | IC2.24 189.56,41.27 188.26,41.27 v185.66,43.87 | IC1.10 148.93,37.7 v150.88,39.65 | IC1.5 146.01,40.95 146.66,41.6 | v147.96,43.87 147.96,42.9 146.66,41.6 | 146.66,41.6 144.06,41.6 | 144.06,41.6 IC1.4 | IC3.10 43.13,37.97 44.11,37 44.11,29.9 | IC3.19 16.66,38.02 16.01,37.37 16.01,29.9 | 44.11,29.9 | 43.96,29.9 44.11,29.9 | IC3.24 20.56,41.27 19.58,41.6 | IC2.3 201.26,42.57 v203.04,43.07 | IC2.4 202.56,41.92 202.88,42.25 | v203.04,43.07 202.88,42.25 | IC2.5 202.56,41.27 202.88,41.6 202.88,42.25 | 126.18,37.7 IC1.19 | IC2.2 199.31,43.22 202.56,43.22 arc90 v203.04,43.07 | v38.43,41.92 IC3.4 | IC3.5 37.78,41.27 v38.43,41.92 | IC3.2 34.85,43.22 35.83,44.52 38.43,44.52 39.08,43.55 39.08,42.57 v38.43,41.92 | IC1.3 143.41,42.25 144.06,41.6 | IC2.10 207.43,38.02 v209.06,39.65 | 125.86,51.67 125.21,51.02 125.21,45.82 130.08,40.95 IC1.24 | IC7.4 64.94,37.64 60.21,37.64 | v89.78,46.47 v86.86,44.52
  Bottom 0.61: 88.16,15.34 ISP1.8 | 90.05,13.65 ISP1.6 | 91.94,11.95 ISP1.4 | IC7.4 IC7.2
  Bottom 0.813: 44.11,29.9 43.96,29.9
  Bottom 1.016: 60.21,29.9 60.21,37.64 v60.21,42.57 | 60.21,29.9 44.11,29.9 | 43.96,29.9 16.01,29.9 2.36,29.9 2.03,30.55 2.03,40.95 2.68,41.6 19.58,41.6 | 109.77,48.59 106.55,47.51 | 106.55,47.51 106.36,47.45 105.59,46.86 101.47,43.79 | 109.77,48.59 113.18,49.72 115.13,51.67 125.86,51.67 | 101.47,43.79 100.51,41.6 99.86,39.65 98.88,35.1 99.53,30.55 | 99.53,30.55 101.81,26.32 | 101.81,26.32 104.41,23.72 v108.63,21.45 v110.58,20.47 115.78,20.47 116.5,20.77 | 116.5,20.77 119.68,22.1 v124.56,27.3 126.18,28.92 126.18,37.7 126.18,38.67 113.83,50.05 | v109.61,51.67 109.61,48.75 109.77,48.59 | 101.81,26.32 | 101.81,26.32 v102.46,25.67 | 88.16,15.34 ISP1.10 85.88,17.22 83.84,18.36 | ISP1.8 90.05,13.65 | ISP1.6 91.94,11.95 | 116.5,20.77 v120.33,10.4 | 79.06,21.12 82.96,18.85 83.84,18.36 | 79.06,21.12 75.81,22.75 72.88,23.4 70.61,23.72 60.21,23.72 60.21,29.9 | 79.06,21.12 v79.06,24.37 | 101.47,43.79 v89.78,46.47 | 99.53,30.55 99.21,30.87 95.96,30.87 91.73,26.65 v91.08,26 88.81,23.73 83.84,18.36 | 125.86,51.67 126.36,51.67 C16.M | v137.56,51.67 125.86,51.67 | ISP2.10 102.3,64.8 105.06,62.4 105.71,61.75 105.71,48.36 106.55,47.51
  other vias: 61.51,26 99.86,40.95
  pour Bottom (isolate 0.508): -0.89,0 226.61,0 227.26,70.2 -0.24,70.2
  pour Top (isolate 0.508): -0.89,0 226.61,0 227.26,70.85 -0.24,70.85
N$1
  Top 1.016: POWER.1 124.29,9.76 D1.A D4.C
N$2
  Top 1.016: POWER.2 129.56,15.18 D3.A 134.63,10.07 132.36,8.12 129.11,6.17 126.51,4.87 123.26,3.57 120.33,2.6 115.78,1.95 112.21,1.62 D2.C D5.A
N$3  (via drill 0.8)
  Top 1.016: 134.57,16.19 IC5.1 131.27,16.9 129.76,16.9 126.72,19.94 C8.2 R18.1 120.98,16.25 119.03,15.27 117.41,14.62 117.41,11.7 C2.+ | 134.57,16.19 136.02,14.75 D3.C | v128.78,12.35 D1.C | v136.26,17.87 135.61,16.9 134.57,16.19
  Bottom 1.016: v128.78,12.35 135.61,16.9 v136.26,17.87
N$5
  Top 0.406: IC8.7 83.61,28.27 83.61,32.17 83.02,32.76 OSZILLATOR.3 81.97,33.46 81.97,37.69 IC6.8
N$6  (via drill 0.61, 0.7)
  Top 0.406: v146.98,45.17 146.33,45.17 145.36,43.87 144.06,41.6 131.71,41.6 v130.41,42.9 | v8.86,44.52 7.01,44.52 R9.1 | 97.4,41.15 97.56,41.15 107,50.6 107,53.95 108.38,55.32 117.67,55.32 v127.27,45.72 | 97.4,41.15 95.88,41.15 94.36,42.51 IC6.21 | v30.04,31.39 33.09,28.34 v64.94,28.34 | v97.4,39.01 97.4,41.15
  Bottom 0.406: IC2.25 189.88,41.92 188.58,43.22 188.58,44.85 188.26,45.17 v146.98,45.17 | IC1.25 131.71,41.6 v130.41,42.9 129.86,43.13 v127.27,45.72 | v8.86,44.52 8.86,43.55 9.51,42.9 20.88,42.9 21.86,41.92 IC3.25 27.3,41.91 27.61,41.91 30.04,39.47 v30.04,31.39 | v64.94,28.34 70.89,28.34 73.63,25.6 79.42,25.6 81.55,23.47 82.77,23.47 91,31.7 91.31,31.7 91.92,32.31 91.92,33.22 89.94,35.2 89.33,35.2 88.72,35.81 88.72,36.73 89.33,37.34 90.24,37.34 91.61,35.96 91.61,35.36 92.22,34.75 93.14,34.75 v97.4,39.01
N$7  (via drill 0.7)
  Top 0.406: v141.46,31.2 141.46,33.23 LED24.C
  Bottom 0.406: IC1.14 141.46,33.44 v141.46,31.2
N$8  (via drill 0.7)
  Top 0.406: v200.93,45.5 202.99,45.5 R1.2
  Bottom 0.406: IC2.1 200.28,43.87 200.93,44.52 v200.93,45.5
N$9
  Top 0.813: C16.P 126.36,63.52 125.21,64.67 123.94,64.67 R2.1
N$10  (via drill 0.7)
  Top 0.406: v165.51,31.2 165.51,33.48 LED17.C
  Bottom 0.406: IC1.6 146.33,40.3 149.58,43.55 160.96,43.55 165.51,39 v165.51,31.2
N$11  (via drill 0.61)
  Top 0.406: v84.91,47.22 83.71,47.22 82.77,46.29 82.77,45.26 81.55,44.04 IC6.2
  Bottom 0.406: v84.91,47.22 84.91,52.73 91.16,58.98 92.38,58.98 93.59,57.76 94.81,57.76 95.73,56.84 97.1,56.84 99.99,59.74 99.99,60.5 ISP2.9
N$12  (via drill 0.61)
  Top 0.406: v77.29,44.65 79.41,42.21 80.63,42.21 80.78,42.2 81.1,42.52 IC6.3 | v58.69,36.57 62.5,36.57 v64.03,35.05 | v88.72,33.37 92.22,36.88 v93.59,36.88 | v96.34,42.21 96.98,45.22 103.54,51.62 103.7,52.36 99.11,57.43 98.47,58.98 ISP2.7
  Bottom 0.406: v77.29,44.65 75.46,44.65 75.15,44.96 73.93,44.96 73.17,44.19 60.22,44.19 58.69,42.67 v58.69,36.57 | v64.03,35.05 65.4,35.05 65.55,35.2 67.84,35.2 69.82,33.22 88.56,33.22 v88.72,33.37 | v93.59,36.88 94.07,37.94 96.34,40.04 v96.34,42.21
N$13
  Top 0.406: IC6.1 79.34,45.6 78.54,46.53 78.73,47.99 86.27,55.02 91.46,54.86 ISP2.1
N$14  (via drill 0.61)
  Top 0.406: v73.17,35.81 71.34,35.81 R4.2 | 87.65,34.29 87.65,36.57 88.88,37.8 IC6.12 | 87.65,34.29 87.65,32.92 87.8,32.76 87.8,31.09 IC8.1 | v87.5,34.29 87.65,34.29
  Bottom 0.406: IC7.3 71.5,35.81 v73.17,35.81 73.63,35.66 74.39,35.66 76.22,33.83 87.04,33.83 v87.5,34.29
N$15  (via drill 0.7)
  Top 0.406: v162.26,31.2 162.26,33.43 LED18.C
  Bottom 0.406: IC1.7 146.66,39.65 149.58,42.57 159.98,42.57 162.26,40.3 v162.26,31.2
N$16  (via drill 0.7)
  Top 0.406: v158.68,31.2 158.68,33.5 LED19.C
  Bottom 0.406: IC1.8 146.98,39 149.58,41.6 157.71,41.6 158.68,40.62 v158.68,31.2
N$17  (via drill 0.7)
  Top 0.406: v155.11,31.2 LED20.C | LED20.C
  Bottom 0.406: IC1.9 147.31,38.35 149.91,40.95 154.46,40.95 155.11,40.3 v155.11,31.2
N$18  (via drill 0.7)
  Top 0.406: v137.56,31.2 137.56,33.53 LED25.C
  Bottom 0.406: IC1.15 135.93,35.1 135.61,34.77 135.61,32.17 v137.56,31.2
N$19  (via drill 0.7)
  Top 0.406: v151.53,31.2 151.53,33.58 LED21.C
  Bottom 0.406: IC1.11 150.88,37.05 151.53,36.07 v151.53,31.2
N$20  (via drill 0.7)
  Top 0.406: v148.28,31.2 148.28,33.4 LED22.C
  Bottom 0.406: IC1.12 147.67,36.36 148.28,35.75 v148.28,31.2
N$21  (via drill 0.7)
  Top 0.406: v144.71,31.2 144.71,33.48 LED23.C
  Bottom 0.406: IC1.13 144.38,35.75 144.71,35.42 v144.71,31.2
N$22  (via drill 0.7)
  Top 0.406: v133.98,31.2 133.98,33.45 LED26.C
  Bottom 0.406: IC1.16 134.63,35.75 133.98,35.1 v133.98,31.2
N$23  (via drill 0.7)
  Top 0.406: v130.41,31.2 130.41,33.38 LED27.C
  Bottom 0.406: IC1.17 131.71,36.4 130.41,35.1 v130.41,31.2
N$24  (via drill 0.7)
  Top 0.406: 127.16,33.2 LED28.C 127.16,33.53 127.16,32.17 v128.46,31.2
  Bottom 0.406: IC1.18 130.08,37.05 128.46,36.4 v128.46,31.2
N$25  (via drill 0.7)
  Top 0.406: LED29.C 123.58,33.55 123.58,31.2 121.43,29.95 110.06,29.95 107.66,32.5 107.66,53.3 108.63,54.6 116.76,54.6 117.46,53.9 v117.46,49.2
  Bottom 0.406: IC1.20 128.46,38.35 122.61,44.2 v117.46,49.2
N$26  (via drill 0.7)
  Top 0.406: v120.66,48.75 120.66,42.9 117.73,40.3 111.23,40.3 109.28,38.35 109.28,32.5 111.21,30.75 119.66,30.75 120.31,31.52 120.33,33.35 LED30.C
  Bottom 0.406: IC1.21 128.78,39 124.56,43.22 120.66,47.45 v120.66,48.75
N$27  (via drill 0.7)
  Top 0.406: v122.28,48.1 122.28,43.22 118.38,39.65 111.88,39.65 110.26,38.02 110.26,33.15 111.51,31.95 116.06,31.95 116.76,32.5 116.76,33.43 LED31.C
  Bottom 0.406: IC1.22 129.43,39.65 122.28,46.8 v122.28,48.1
N$28  (via drill 0.7)
  Top 0.406: v123.91,47.12 123.91,43.55 122.93,42.57 118.71,39 112.21,39 111.23,38.02 111.23,33.8 111.88,33.15 112.68,33.15 LED32.C
  Bottom 0.406: IC1.23 129.76,40.3 123.91,46.15 v123.91,47.12
N$29  (via drill 0.7)
  Top 0.406: v144.22,44.52 R6.2
  Bottom 0.406: IC1.1 143.41,43.55 v144.22,44.52
N$30  (via drill 0.61)
  Top 0.406: v87.19,26.36 87.19,24.08 86.28,23.16 IC8.12 | 90.85,33.83 90.39,33.83 89.78,33.22 89.78,30.48 IC8.32 | 90.85,33.83 91.31,33.83 91.92,33.22 91.92,32.61 92.53,32 v92.53,31.39 92.98,31.24 95.88,28.34 101.37,28.34 103.65,26.06 103.65,23.47 101.82,21.64 101.82,21.03 R13.2 | v91.46,37.64 91.46,38.56 90.7,39.32 IC6.15 | v92.68,35.81 90.85,33.98 90.85,33.83
  Top 1.016: 104.55,14.78 R5.2 | 104.55,14.78 104.73,14.95 | 104.55,14.78 104.54,14.78 D6.3 101.66,18.02 100.83,18.85 R13.2
  Bottom 0.406: v87.19,26.36 92.22,31.39 v92.53,31.39 | v91.46,37.64 91.46,37.03 v92.68,35.81
N$31
  Top 1.016: D5.C arc90 104.17,7.99 R5.1
N$33  (via drill 0.61)
  Top 0.406: C1.2 96.64,16.76 97.25,16.15 R14.1 96.49,14.93 94.81,13.26 ISP1.5 | v95.88,25.6 95.88,26.67 92.98,29.56 92.53,29.56 92.38,29.41 92.22,29.41 IC8.29
  Bottom 0.406: v95.88,25.6 95.88,14.78 94.66,13.56 ISP1.5
N$34  (via drill 0.7)
  Top 0.406: v56.11,31.5 LED33.C | LED33.C
  Bottom 0.406: IC3.6 54.36,40.62 56.11,39 v56.11,31.5
N$35  (via drill 0.7)
  Top 0.406: v52.61,31.5 LED34.C | LED34.C
  Bottom 0.406: IC3.7 50.13,39.97 52.61,37.5 v52.61,31.5
N$36  (via drill 0.7)
  Top 0.406: v49.11,31.5 LED35.C | LED35.C
  Bottom 0.406: IC3.8 46.56,39.32 49.11,37 v49.11,31.5
N$37  (via drill 0.7)
  Top 0.406: v45.61,31.5 LED36.C | LED36.C
  Bottom 0.406: IC3.9 44.48,38.62 45.61,37.5 v45.61,31.5
N$38  (via drill 0.7)
  Top 0.406: v42.11,31.5 LED37.C | LED37.C
  Bottom 0.406: IC3.11 41.03,37.37 42.11,36.5 v42.11,31.5
N$39  (via drill 0.7)
  Top 0.406: v38.61,31.5 LED38.C | LED38.C
  Bottom 0.406: IC3.12 37.46,36.72 38.61,36 v38.61,31.5
N$40  (via drill 0.7)
  Top 0.406: v35.11,31.5 LED39.C | LED39.C
  Bottom 0.406: IC3.13 34.58,36.02 35.11,35.5 v35.11,31.5
N$41  (via drill 0.7)
  Top 0.406: v221.41,31.2 221.41,33.38 LED1.C
  Bottom 0.406: IC2.6 203.53,40.62 207.11,43.87 217.51,43.87 221.41,39.32 v221.41,31.2
N$42  (via drill 0.7)
  Top 0.406: v218.16,31.2 218.16,33.53 LED2.C
  Bottom 0.406: IC2.7 204.18,39.97 207.43,42.9 216.21,42.9 218.16,40.62 v218.16,31.2
N$43  (via drill 0.7)
  Top 0.406: v214.58,31.2 214.58,33.55 LED3.C
  Bottom 0.406: IC2.8 204.83,39.32 207.76,41.92 213.28,41.92 214.58,40.62 v214.58,31.2
N$44  (via drill 0.7)
  Top 0.406: v211.01,31.2 211.01,33.48 LED4.C
  Bottom 0.406: IC2.9 205.48,38.67 208.08,40.95 210.68,40.95 211.01,40.62 v211.01,31.2
N$45  (via drill 0.7)
  Top 0.406: v207.76,31.2 207.76,33.43 LED5.C
  Bottom 0.406: IC2.11 207.11,37.37 207.76,36.72 v207.76,31.2
N$46  (via drill 0.7)
  Top 0.406: v204.18,31.2 204.18,33.5 LED6.C
  Bottom 0.406: IC2.12 203.53,36.72 204.18,36.07 v204.18,31.2
N$47  (via drill 0.7)
  Top 0.406: v200.61,31.2 LED7.C
  Bottom 0.406: IC2.13 200.76,36.07 200.93,35.59 200.93,31.52 v200.61,31.2
N$48  (via drill 0.7)
  Top 0.406: v197.03,31.2 197.03,32.82 LED8.C
  Bottom 0.406: IC2.14 197.36,35.42 197.03,35.1 v197.03,31.2
N$49  (via drill 0.7)
  Top 0.406: v193.46,31.2 193.46,33.58 LED9.C
  Bottom 0.406: IC2.15 193.46,35.4 v193.46,31.2
N$50  (via drill 0.7)
  Top 0.406: v189.88,31.2 189.88,33.35 LED10.C
  Bottom 0.406: IC2.16 190.53,36.07 189.88,35.42 v189.88,31.2
N$51  (via drill 0.7)
  Top 0.406: v186.63,31.2 186.63,33.55 LED11.C
  Bottom 0.406: IC2.17 187.28,36.72 186.63,36.07 v186.63,31.2
N$52  (via drill 0.7)
  Top 0.406: v183.06,31.2 183.06,33.53 LED12.C
  Bottom 0.406: IC2.18 184.03,37.37 183.06,36.4 v183.06,31.2
N$53  (via drill 0.7)
  Top 0.406: v179.81,31.2 179.81,33.38 LED13.C
  Bottom 0.406: IC2.20 185.33,38.67 183.06,40.95 180.78,40.95 179.81,39.65 v179.81,31.2
N$54  (via drill 0.7)
  Top 0.406: v176.23,31.2 176.23,33.45 LED14.C
  Bottom 0.406: IC2.21 185.98,39.32 183.38,41.92 177.86,41.92 176.23,39.97 v176.23,31.2
N$55  (via drill 0.7)
  Top 0.406: v172.66,31.2 172.66,33.53 LED15.C
  Bottom 0.406: IC2.22 186.63,39.97 183.71,42.9 175.26,42.9 172.66,39.97 v172.66,31.2
N$56  (via drill 0.7)
  Top 0.406: v169.08,31.2 169.08,33.55 LED16.C
  Bottom 0.406: IC2.23 187.28,40.62 184.03,43.87 172.01,43.87 169.08,40.95 v169.08,31.2
N$57  (via drill 0.61)
  Top 0.406: R3.2 C12.2 98.32,55.93 96.64,57.61 ISP2.5 | v83.84,45.83 83.84,44.19 82.62,42.98 IC6.4
  Bottom 0.406: v83.84,45.83 83.84,52.58 91.77,60.5 94.2,60.5 96.03,58.67 ISP2.5
N$58  (via drill 0.7)
  Top 0.406: v31.61,31.5 LED40.C | LED40.C
  Bottom 0.406: v31.61,31.5 33.21,32.12 33.23,32.15 33.23,35.1 32.91,35.42 IC3.14
N$59  (via drill 0.7)
  Top 0.406: v28.11,31.5 LED41.C | LED41.C
  Bottom 0.406: IC3.15 26.41,35.42 26.08,35.1 26.08,33.52 v28.11,31.5
N$60  (via drill 0.7)
  Top 0.406: v24.61,31.5 LED42.C | LED42.C
  Bottom 0.406: IC3.16 25.11,36.07 24.61,35.5 v24.61,31.5
N$61  (via drill 0.7)
  Top 0.406: v21.21,31.52 LED43.C
  Bottom 0.406: IC3.17 22.18,36.72 21.21,35.75 v21.21,31.52
N$62  (via drill 0.7)
  Top 0.406: v17.61,31.5 LED44.C
  Bottom 0.406: IC3.18 17.96,37.37 17.61,37 v17.61,31.5
N$63  (via drill 0.7)
  Top 0.406: v14.11,31.5 LED45.C
  Bottom 0.406: IC3.20 15.03,38.67 14.11,38 v14.11,31.5
N$64  (via drill 0.7)
  Top 0.406: v10.61,31.5 LED46.C
  Bottom 0.406: IC3.21 11.13,39.32 10.61,38.5 v10.61,31.5
N$65  (via drill 0.7)
  Top 0.406: v7.11,31.5 LED47.C
  Bottom 0.406: IC3.22 7.56,39.97 7.11,39.5 v7.11,31.5
N$66  (via drill 0.7)
  Top 0.406: v3.61,31.5 LED48.C
  Bottom 0.406: IC3.23 4.63,40.62 3.61,39.5 v3.61,31.5
N$67  (via drill 0.7)
  Top 0.406: v34.37,44.52 41.36,44.52 arc-15 R10.2
  Bottom 0.406: IC3.1 33.88,43.87 v34.37,44.52
N$68  (via drill 0.61)
  Top 0.406: v104.26,58.82 107.92,62.48 R11.2 | IC6.31 90.7,51.36 v92.07,52.73 | v115.84,64.16 114.17,64.16 T1.E
  Top 0.61: R11.2 112.11,63.2 arc90 T1.E
  Bottom 0.406: v92.07,52.73 98.17,52.73 v104.26,58.82 | v115.84,64.16 114.17,64.16 T2.E
N$69  (via drill 0.61)
  Top 0.406: v74.24,30.02 70.73,30.02 69.96,29.99 69.52,30.63 R12.2
  Bottom 0.406: v74.24,30.02 69.21,30.02 D7.C
N$70  (via drill 0.61)
  Top 0.406: v84.75,32.15 84.75,35.05 87.19,37.49 87.19,38.56 88.56,39.93 89.02,39.93 89.17,39.77 IC6.14 | v74.09,26.67 70.58,26.67 69.52,27.74 R12.1
  Bottom 0.406: v84.75,32.15 79.57,32.15 v74.09,26.67
N$71  (via drill 0.61)
  Top 0.406: v87.19,18.13 87.03,19.94 87.03,20.25 IC8.15
  Bottom 0.406: v87.19,18.13 93.9,11.43 94.51,11.43 96.03,9.9 97.56,9.9 ISP1.1
N$72
  Top 0.406: 72.18,28.53 R15.1 72.87,28.5 75.76,28.5 OSZILLATOR.1
N$73  (via drill 0.61)
  Top 0.406: v89.78,18.59 90.55,19.35 90.55,20.12 IC8.17
  Bottom 0.406: v89.78,18.59 90.09,18.59 92.22,16.46 92.22,15.24 ISP1.7
N$74
  Top 0.406: IC8.16 88.11,19.96 88.11,18.74 90.09,16.76 ISP1.9
N$75
  Top 0.406: LED50.C 100.76,33.53 99.38,33.53 R17.2
N$76
  Top 0.406: LED49.C 103.96,32.76 101.98,30.78 R16.2
N$77
  Top 0.406: IC6.16 91.46,39.77 93.44,37.95 94.05,37.95 95.12,36.88 95.12,34.9 R17.1
N$78  (via drill 0.61)
  Top 0.406: v89.78,36.27 89.63,36.42 89.63,38.25 IC6.13 | v93.44,32.61 94.66,32.61 96.49,30.78 98.78,30.78 R16.1
  Bottom 0.406: v93.44,32.61 v89.78,36.27
N$79  (via drill 0.61)
  Top 0.406: v82.01,24.53 82.47,24.08 83.69,23.92 IC8.9 | v86.13,32 v86.13,34.9 | v83.68,35.96 85.35,37.79 IC6.11
  Bottom 0.406: v82.01,24.53 82.01,27.89 v86.13,32 | v86.13,34.9 84.91,34.9 v83.68,35.96
RXD  (via drill 0.61)
  Top 0.406: v86.56,41.99 86.13,40.69 85.36,39.93 IC6.9 | v75.46,39.93 75.46,42.52 76.22,43.28 76.22,45.41 75.76,45.87 RS232.1
  Bottom 0.406: v86.56,41.99 86.28,40.69 85.52,39.93 v75.46,39.93
SCL  (via drill 0.61, 0.7)
  Top 0.406: v14.71,44.52 12.43,44.52 R8.1 | v128.8,29.26 109.75,29.26 107,32 107,36.42 105.63,37.79 96.95,37.79 v94.36,40.22 93.35,41.28 IC6.19 | v52.75,41.76 53.82,41.76 54.27,42.21 58.85,42.21 59.61,41.45 v64.94,41.45
  Bottom 0.406: IC2.26 190.21,42.57 189.23,43.55 189.23,45.5 188.91,45.82 148.93,45.82 147.63,47.12 141.31,47.12 140.71,46.56 140.71,45.12 139.41,43.82 139.41,42.24 | IC3.26 22.51,42.57 20.56,44.52 | v14.71,44.52 20.56,44.52 | v128.8,29.26 138.45,29.26 139.41,30.85 139.41,42.24 | v52.75,41.76 48.79,45.72 21.97,45.72 20.75,44.5 20.56,44.52 | v64.94,41.45 71.95,41.45 72.41,40.99 83.39,40.99 85.09,42.69 85.09,42.76 85.56,43.22 91.08,43.22 91.73,42.9 92.05,42.53 v94.36,40.22 | 139.41,42.24 135.59,42.24 IC1.26
SDA  (via drill 0.61, 0.7)
  Top 0.406: R7.1 17.53,43.55 20.23,43.55 21.21,44.52 v22.51,44.52 23.03,44.65 25.01,46.63 72.11,46.63 72.41,46.94 73.48,46.94 74.24,46.18 74.24,44.65 73.63,44.04 73.63,42.98 74.09,42.52 v74.09,39.77 | v98.03,47.96 97.55,47.51 94.84,44.96 92.14,44.8 91.72,44.22 92.2,43.6 92.67,43.13 IC6.20 | v127.27,48.77 120.11,55.93 108.07,55.93 105.03,53.12 104.71,51.48 v100.74,47.16 100.75,45.9 99.31,44.3 v97.71,42.82 | v88.26,41.95 88.26,42.82 v88.62,44.41
  Bottom 0.406: IC2.27 190.53,43.22 189.88,43.87 189.88,46.15 189.56,46.47 149.26,46.47 147.96,47.77 133.98,47.77 133.01,46.8 | 133.01,46.8 133.01,43.55 133.66,42.9 IC1.27 | IC3.27 23.81,43.22 v22.51,44.52 | v100.74,47.16 v98.03,47.96 | v127.27,48.77 131.08,48.77 132.91,46.94 133.01,46.8 | v74.09,39.77 75,38.86 86.58,38.86 88.26,40.54 v88.26,41.95 | v97.71,42.82 96.33,43.55 91.41,44.52 88.92,44.41 v88.62,44.41
TXD  (via drill 0.61)
  Top 0.406: v90.85,32.76 91.31,32.31 91.31,30.78 91.16,30.63 91.16,30.48 IC8.31 | v83.53,37.5 84.91,38.4 IC6.10 | v58.54,35.2 v62.35,35.2 | v73.78,34.44 v75.3,36.6
  Bottom 0.406: v90.85,32.76 86.28,37.34 v83.53,37.5 83.23,37.66 82.16,36.6 v75.3,36.6 | v58.54,35.2 57.63,36.12 57.63,42.52 59.91,44.8 69.82,44.8 71.95,46.94 73.76,47.1 74.21,47.23 75.15,47.55 75.46,47.7 76.4,48.02 78.35,45.26 78.35,44.19 77.74,43.58 75.61,43.58 RS232.2 | v62.35,35.2 62.66,35.2 63.57,36.12 64.49,36.12 64.79,35.81 68.14,35.81 69.52,34.44 v73.78,34.44

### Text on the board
Bottom: Coll | T2 | IC3 | Pin1 | IC1 | IC2 | Pin1 | 1 | 1 | 1 | IC7 | CATH | D7 | Propelleruhr Projekt von Robotikhardware.de | Nicht ohne Propellerschutz (z.B. Haube) betreiben
tPlace: 1 | TTL | 1 | Anoden | Anoden | Anoden | PropellerClock | Roboternetz | Version 1 Rev.12 Projekt www.mikrocontroller-elektronik.de | Hochauflösend mit 50 dimmbaren LEDs und zwei Controllern | ~ | ~ | 1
